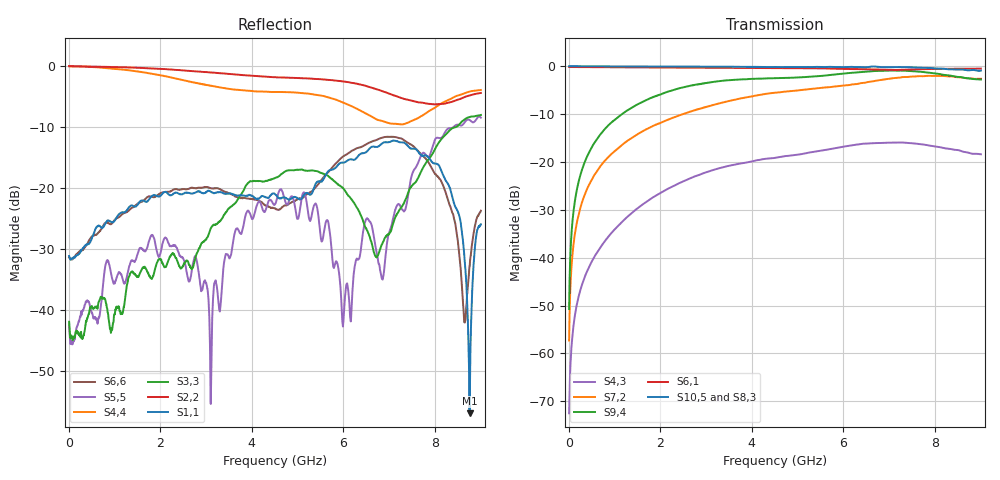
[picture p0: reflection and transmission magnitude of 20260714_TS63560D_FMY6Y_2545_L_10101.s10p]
# GHz S DB R 50
! CMT, SN0916, 25263762, 26.7.0
! Date: 15.07.2026 13:44:55
! Data: Format
! Freq S1.1:dB/Ang S1.2:dB/Ang S1.3:dB/Ang S1.4:dB/Ang S1.5:dB/Ang S1.6:dB/Ang S1.7:dB/Ang S1.8:dB/Ang S1.9:dB/Ang S1.10:dB/Ang
!  S2.1:dB/Ang S2.2:dB/Ang S2.3:dB/Ang S2.4:dB/Ang S2.5:dB/Ang S2.6:dB/Ang S2.7:dB/Ang S2.8:dB/Ang S2.9:dB/Ang S2.10:dB/Ang
!  S3.1:dB/Ang S3.2:dB/Ang S3.3:dB/Ang S3.4:dB/Ang S3.5:dB/Ang S3.6:dB/Ang S3.7:dB/Ang S3.8:dB/Ang S3.9:dB/Ang S3.10:dB/Ang
!  S4.1:dB/Ang S4.2:dB/Ang S4.3:dB/Ang S4.4:dB/Ang S4.5:dB/Ang S4.6:dB/Ang S4.7:dB/Ang S4.8:dB/Ang S4.9:dB/Ang S4.10:dB/Ang
!  S5.1:dB/Ang S5.2:dB/Ang S5.3:dB/Ang S5.4:dB/Ang S5.5:dB/Ang S5.6:dB/Ang S5.7:dB/Ang S5.8:dB/Ang S5.9:dB/Ang S5.10:dB/Ang
!  S6.1:dB/Ang S6.2:dB/Ang S6.3:dB/Ang S6.4:dB/Ang S6.5:dB/Ang S6.6:dB/Ang S6.7:dB/Ang S6.8:dB/Ang S6.9:dB/Ang S6.10:dB/Ang
!  S7.1:dB/Ang S7.2:dB/Ang S7.3:dB/Ang S7.4:dB/Ang S7.5:dB/Ang S7.6:dB/Ang S7.7:dB/Ang S7.8:dB/Ang S7.9:dB/Ang S7.10:dB/Ang
!  S8.1:dB/Ang S8.2:dB/Ang S8.3:dB/Ang S8.4:dB/Ang S8.5:dB/Ang S8.6:dB/Ang S8.7:dB/Ang S8.8:dB/Ang S8.9:dB/Ang S8.10:dB/Ang
!  S9.1:dB/Ang S9.2:dB/Ang S9.3:dB/Ang S9.4:dB/Ang S9.5:dB/Ang S9.6:dB/Ang S9.7:dB/Ang S9.8:dB/Ang S9.9:dB/Ang S9.10:dB/Ang
!  S10.1:dB/Ang S10.2:dB/Ang S10.3:dB/Ang S10.4:dB/Ang S10.5:dB/Ang S10.6:dB/Ang S10.7:dB/Ang S10.8:dB/Ang S10.9:dB/Ang S10.10:dB/Ang
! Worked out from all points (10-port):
!   2001 points, 10 MHz to 9 GHz, reference 50 ohm
!   strongest paths, dB at 10 MHz, 2.257 GHz, 4.505 GHz, 6.753 GHz, 9 GHz:
!     S10,5: -0.1, -0.2, -0.2, -0.2, -1.0
!     S8,3: -0.1, -0.2, -0.4, -0.4, -1.3
!     S6,1: -0.2, -0.4, -0.5, -0.8, -0.6
!     S9,4: -50.7, -5.1, -2.6, -1.1, -2.9
!     S7,2: -57.3, -10.9, -5.6, -3.0, -2.7
!     S4,3: -72.5, -25.2, -19.2, -16.1, -18.4
!   lowest |S11| = -56.9 dB at 8.753 GHz (marker M1), VSWR 1.00, Z = 50 - j0.143 ohm
!   |S11| at or under -10 dB: start of sweep to end of sweep
